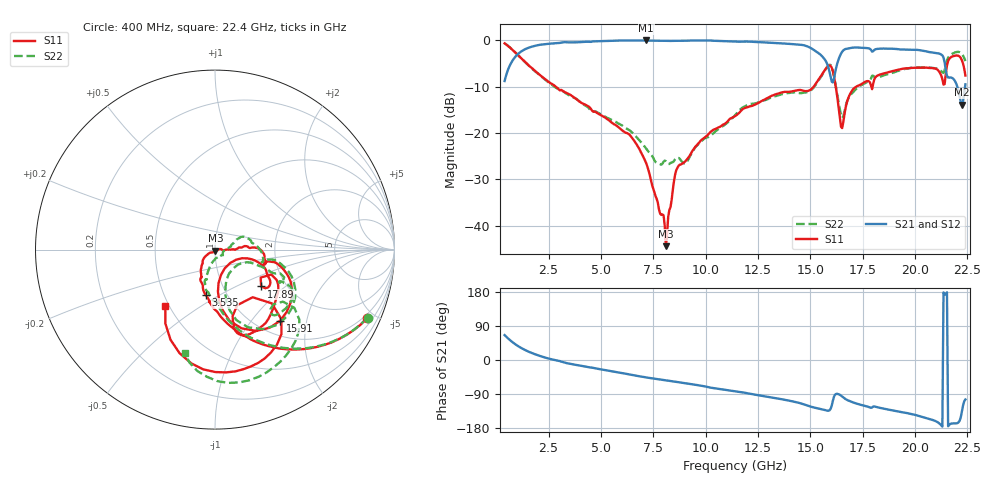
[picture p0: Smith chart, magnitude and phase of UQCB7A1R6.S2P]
!  Part Number  UQCB7A1R6	Mounting Orientation: Vertical
!  Description: RF capacitors
!  Application: Coupling, Bypass, Tuning, DC Block
!  Filters, Matching
# GHZ S DB R 50
! Freq  |S11|  S11 Ph  |S21|  S21 Ph  |S12|  S12 Ph  |S22|  S22 Ph
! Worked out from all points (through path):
!   401 points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, 400 MHz to 22.4 GHz, reference 50 ohm
!   highest |S21| = 0.00 dB at 7.165 GHz (marker M1); lowest = -13.8 dB at 22.23 GHz (marker M2)
!   group delay of S21, straight-line fit = 24.1 ps
!   lowest |S11| = -44.4 dB at 8.1 GHz (marker M3), VSWR 1.01, Z = 50.2 - j0.56 ohm
!   |S11| at or under -10 dB: 2.843 GHz to 15.15 GHz (12.31 GHz wide, 137 % of centre); 16.21 GHz to 17.18 GHz (973.3 MHz wide, 5.83 % of centre); 17.91238 GHz to 17.96818 GHz (55.8 MHz wide, 0.311 % of centre)
!   |S22| runs from -26.8 to -0.6 dB; largest |S21 - S12| = 0.0032
!   S11 on the Smith chart (normalised r, x): 400 MHz: 0.80, -4.50; 3.535 GHz: 0.80, -0.43; 15.91 GHz: 1.27, -1.41; 17.89 GHz: 1.50, -0.69; 22.4 GHz: 0.48, -0.36
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0.4  -0.64 -24.4  -8.76 65.7  -8.76 65.7  -0.62 -24.0
1.61  -5.64 -69.5  -1.48 20.4  -1.48 20.5  -5.64 -68.5
3.535  -11.72 -101.5  -0.42 -10.2  -0.42 -10.1  -11.97 -97.2
4.085  -13.51 -108.8  -0.34 -15.6  -0.33 -15.6  -13.54 -104.9
6.395  -20.50 -137.1  -0.01 -38.5  -0.01 -38.5  -19.50 -107.3
7.165  -26.55 -147.4  0.00 -46.0  -0.01 -46.0  -23.32 -100.4
7.77  -36.45 -118.9  -0.07 -51.1  -0.07 -51.1  -26.59 -73.1
8.1  -44.40 -67.8  -0.08 -53.8  -0.08 -53.8  -26.08 -58.6
8.705  -27.05 -6.8  -0.09 -58.6  -0.08 -58.6  -25.35 -35.0
11.4  -16.34 5.0  -0.25 -82.6  -0.25 -82.6  -16.15 26.0
15.085  -10.34 -12.5  -1.83 -124.2  -1.81 -124.0  -10.51 -10.7
15.91  -5.39 -47.4  -6.72 -132.9  -6.70 -133.0  -5.24 -43.1
16.185  -9.34 -82.7  -6.82 -90.9  -6.80 -90.9  -9.15 -76.4
16.515  -18.92 -40.9  -2.45 -96.2  -2.46 -96.3  -16.71 -46.1
17.01  -10.69 -19.8  -1.55 -111.3  -1.55 -111.4  -11.29 -20.1
17.89  -9.65 -38.6  -2.01 -126.2  -2.01 -126.2  -8.23 -20.1
18.77  -6.80 -44.3  -1.79 -131.3  -1.76 -131.3  -7.19 -25.8
21.19  -7.06 -76.3  -2.91 -169.1  -2.90 -169.1  -6.46 -48.7
21.41  -9.41 -51.7  -4.78 173.2  -4.77 173.2  -6.43 -37.4
21.63  -3.97 -57.0  -8.02 -170.7  -8.02 -170.7  -3.38 -48.4
22.235  -4.30 -109.0  -13.84 -135.6  -13.86 -135.6  -2.97 -93.5
22.4  -7.56 -131.3  -9.47 -104.2  -9.46 -104.2  -4.45 -106.5
